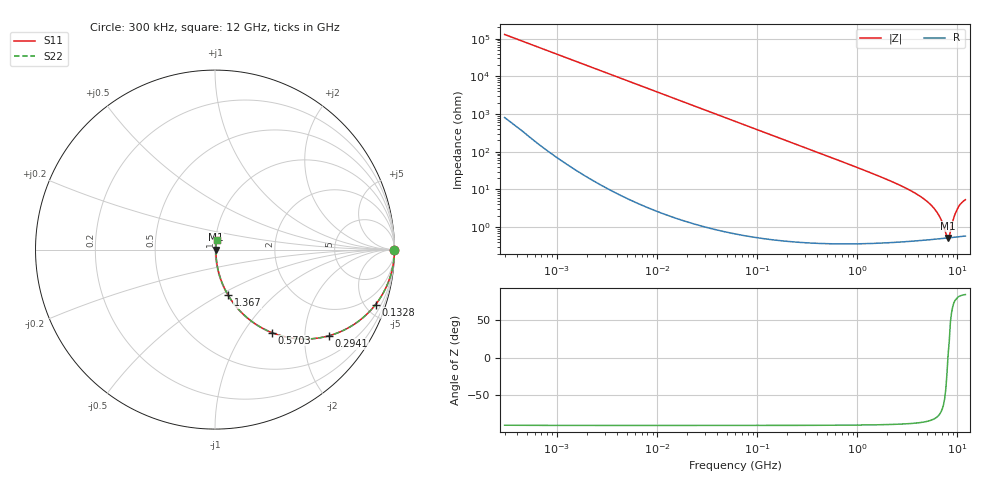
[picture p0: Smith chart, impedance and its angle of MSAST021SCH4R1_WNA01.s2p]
! MSAST021SCH4R1_WNA01  S-PARAMETER MODEL  ( General Type )
! Model Generated by TAIYO YUDEN Corporation (http://www.ty-top.com)
! Version 2.0
! TAIYO YUDEN Control No. 181101
! Copyright(c) 2015 TAIYO YUDEN CO.,LTD. All Rights Reserved.
! Product Description (link to TY-COMPAS)
! https://ds.yuden.co.jp/TYCOMPAS/or/detail?pn=MSAST021SCH4R1BWNA01&u=M
! Products Name : Multilayer Ceramic Capacitors
! Characteristics :
!  Capacitance : 4.1 pF , Rated Voltage : 25V , TCC : CH / C0H
!  Case Size : 0.25 x 0.125 / 0.0098 x 0.0049 [mm/inch] , Thickness : 0.125 / 0.0049 [mm/inch]
!  (Conditions: Temperature = 25 degC , DC Bias Current/Voltage = 0A / 0V)
! External Node Assignments :
!  1  o---| |---o  2
! GND o---------o GND
! Frequency Range : 0.3MHz  -  12000MHz  [ 401 STEP ]
# MHz S RI R 50
! Freq[MHz].  S11 Real  S11 Imag  S21 Real  S21 Imag  S12 Real  S12 Imag  S22 Real  S22 Imag
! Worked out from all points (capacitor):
!   401 points, 300 kHz to 12 GHz, reference 50 ohm
!   read as one part in series: C = 4.1 pF near 316.3 kHz
!   lowest |Z| = 521 mohm at 8.065 GHz (marker M1)
!   series resonance near 8.032 GHz, so ESL is about 96 pH
!   S11 on the Smith chart (normalised r, x): 300 kHz: open; 132.8 MHz: 1.01, -5.84; 294.1 MHz: 1.01, -2.64; 570.3 MHz: 1.01, -1.35; 1.367 GHz: 1.01, -0.55; 12 GHz: 1.01, +0.11
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0.3  1 -0.000773  5.44e-06 0.000773  5.44e-06 0.000773  1 -0.000773
1.769972  1 -0.00456  2.62e-05 0.00456  2.62e-05 0.00456  1 -0.00456
10.44266  0.9993 -0.0269  0.000741 0.0269  0.000741 0.0269  0.9993 -0.0269
60  0.9765 -0.1509  0.0235 0.1509  0.0235 0.1509  0.9765 -0.1509
132.8329  0.8947 -0.3061  0.1053 0.3061  0.1053 0.3061  0.8947 -0.3061
294.0765  0.6344 -0.4801  0.3656 0.4801  0.3656 0.4801  0.6344 -0.4801
353.9943  0.5448 -0.4963  0.4552 0.4963  0.4552 0.4963  0.5448 -0.4963
570.2811  0.3154 -0.462  0.6846 0.462  0.6846 0.462  0.3154 -0.462
871.3074  0.1644 -0.3666  0.8356 0.3666  0.8356 0.3666  0.1644 -0.3666
1366.97  0.0736 -0.2545  0.9264 0.2545  0.9264 0.2545  0.0736 -0.2545
2088.533  0.0327 -0.1669  0.9673 0.1669  0.9673 0.1669  0.0327 -0.1669
3642.919  0.0113 -0.0832  0.9887 0.0832  0.9887 0.0832  0.0113 -0.0832
5278.635  0.00634 -0.0412  0.9937 0.0412  0.9937 0.0412  0.00634 -0.0412
6524.734  0.00528 -0.0199  0.9947 0.0199  0.9947 0.0199  0.00528 -0.0199
7064.448  0.00514 -0.0122  0.9949 0.0122  0.9949 0.0122  0.00514 -0.0122
7648.807  0.00512 -0.00451  0.9949 0.00451  0.9949 0.00451  0.00512 -0.00451
8064.993  0.00517 0.000359  0.9948 -0.000359  0.9948 -0.000359  0.00517 0.000359
8503.825  0.00528 0.00567  0.9947 -0.00567  0.9947 -0.00567  0.00528 0.00567
9207.246  0.00566 0.0171  0.9943 -0.0171  0.9943 -0.0171  0.00566 0.0171
9968.853  0.00635 0.0293  0.9937 -0.0293  0.9937 -0.0293  0.00635 0.0293
10793.46  0.00733 0.0413  0.9927 -0.0413  0.9927 -0.0413  0.00733 0.0413
12000  0.00858 0.0526  0.9914 -0.0526  0.9914 -0.0526  0.00858 0.0526
